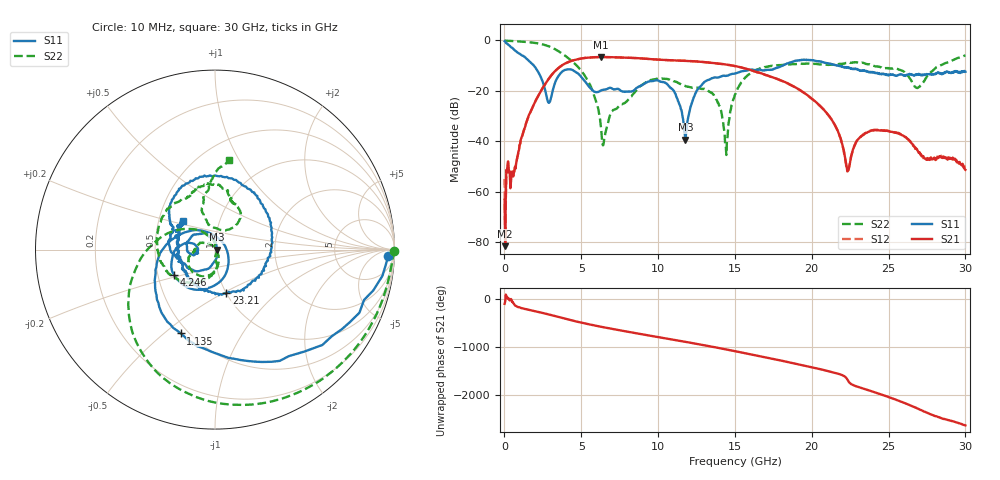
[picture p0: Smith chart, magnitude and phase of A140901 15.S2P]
!  2-Port S-parameters saved by WinCal
! VAR MeasName=S-Parameters (CALIBRATED_DATA) read from VNA (N5244A)
! VAR MeasDate=11/3/2014 9:27:55 AM
! VAR NAME=A140901 15
! VAR FILENAME=A140901 15.S2P
! VAR DATE=11/3/2014 9:27:55 AM
! VAR PHYS_PORTS=1,2
# Hz S RI R 50
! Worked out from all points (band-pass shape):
!   801 points, 10 MHz to 30 GHz, reference 50 ohm
!   highest |S21| = -6.56 dB at 6.27 GHz (marker M1); lowest = -81.5 dB at 47.49 MHz (marker M2)
!   |S21| within 3 dB of the highest: 3.825 GHz to 14.42 GHz (10.59 GHz wide, 116 % of centre)
!   lowest |S11| = -39.4 dB at 11.78 GHz (marker M3), VSWR 1.02, Z = 51.1 - j0.0153 ohm
!   |S11| at or under -10 dB: 1.919 GHz to 18.11 GHz (16.19 GHz wide, 162 % of centre); 21.67 GHz to end of sweep
!   |S22| runs from -45.4 to 0.0 dB; largest |S21 - S12| = 0.0045
!   S11 on the Smith chart (normalised r, x): 10 MHz: 25, -29; 1.135 GHz: 0.46, -0.57; 4.246 GHz: 0.61, -0.18; 23.21 GHz: 1.00, -0.52; 30 GHz: 0.67, +0.23
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1e7  0.9654 -0.038  -0.000159 -0.000679  0.00167 0.000678  0.9977 -0.00775
4.74875e7  0.933 -0.1459  4.73e-05 -6.94e-05  6.34e-05 0.000102  0.9929 -0.0366
1.134625e9  -0.1906 -0.4669  -0.0119 0.00311  -0.012 0.00321  0.7066 -0.6315
2.896538e9  0.0474 0.0333  0.1466 0.0988  0.1462 0.0989  -0.3069 -0.6991
4.246088e9  -0.2293 -0.1396  0.0718 -0.3761  0.0719 -0.3758  -0.4188 -0.0594
5.033325e9  -0.1814 0.0284  -0.328 -0.2937  -0.3281 -0.2935  -0.2188 0.1063
6.270412e9  -0.101 -0.0129  -0.352 0.311  -0.3519 0.3106  0.00327 0.0199
8.332225e9  -0.0959 -0.0221  0.4334 0.1238  0.4326 0.1238  0.0123 -0.0829
1.001916e10  -0.1539 0.0446  0.0799 -0.4094  0.0789 -0.4081  -0.1179 -0.1324
1.178108e10  0.0107 -0.00015  -0.3944 -0.0158  -0.3951 -0.0159  -0.1237 -0.0172
1.249334e10  -0.0245 -0.0943  -0.296 0.243  -0.2971 0.2433  -0.1162 -0.00462
1.358048e10  -0.148 -0.1045  0.084 0.3475  0.086 0.3465  -0.0759 0.0386
1.44052e10  -0.188 -0.0632  0.3003 0.1438  0.3005 0.1408  0.00474 0.0064
1.5005e10  -0.2174 -0.0402  0.3031 -0.0681  0.3011 -0.0714  0.0184 -0.0827
1.721676e10  -0.2348 0.1122  -0.1813 -0.0773  -0.1806 -0.0767  -0.3 -0.074
2.002832e10  0.0953 0.3963  0.0683 0.00919  0.0682 0.00971  -0.2392 0.2429
2.152782e10  0.319 0.0677  -0.00605 -0.0197  -0.006 -0.0196  -0.1432 0.2963
2.231506e10  0.2592 -0.1363  -0.00112 0.00229  -0.00105 0.00237  -0.0998 0.3458
2.321476e10  0.0638 -0.2414  0.00578 -0.0111  0.00562 -0.0114  0.0148 0.3603
2.501416e10  -0.1639 -0.1195  -0.00431 0.0153  -0.00413 0.0155  0.0991 0.2653
2.688854e10  -0.2134 -0.000907  -0.00448 -0.00477  -0.0046 -0.00493  0.0243 0.1117
3e10  -0.1769 0.1607  -0.00162 -0.0022  -0.00154 -0.00222  0.0764 0.4984
